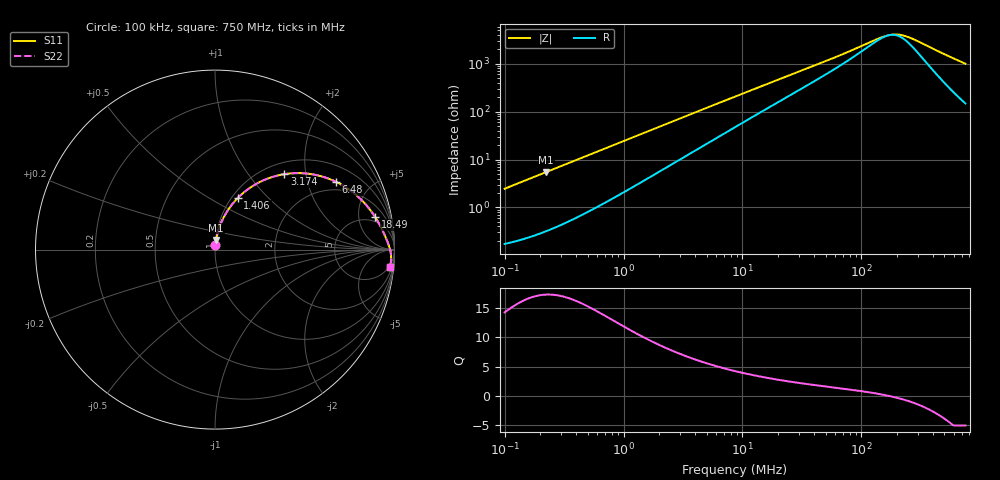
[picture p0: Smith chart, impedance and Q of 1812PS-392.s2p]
# MHz S MA R 50
!Freq  MagS11  AngS11  MagS21  AngS21  MagS12  AngS12  MagS22  AngS22
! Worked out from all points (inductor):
!   801 points, 100 kHz to 750 MHz, reference 50 ohm
!   read as one part in series: L = 3.89 uH near 104.6 kHz
!   highest Q = 17.2 at 223.2 kHz (marker M1), where L = 3.89 uH
!   self-resonance near 172.1 MHz
!   S11 on the Smith chart (normalised r, x): 100 kHz: 1.00, +0.05; 1.406 MHz: 1.07, +0.68; 3.174 MHz: 1.22, +1.52; 6.48 MHz: 1.62, +3.05; 18.49 MHz: 3.84, +8.16; 750 MHz: 4, -20
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0.1  0.02448 84.6  0.998 -1.4  0.998 -1.4  0.02448 84.6
0.2232315  0.05441 83.6  0.9954 -3.1  0.9954 -3.1  0.05441 83.6
0.4457309  0.1076 80.2  0.9874 -6.2  0.9874 -6.2  0.1076 80.2
0.8511669  0.2003 74.0  0.9641 -11.5  0.9641 -11.5  0.2003 74.0
1.406005  0.3148 66.1  0.9189 -18.3  0.9189 -18.3  0.3148 66.1
1.964725  0.4132 59.2  0.8649 -24.2  0.8649 -24.2  0.4132 59.2
2.539275  0.497 53.1  0.8064 -29.5  0.8064 -29.5  0.497 53.1
3.173849  0.5715 47.4  0.7432 -34.4  0.7432 -34.4  0.5715 47.4
4.484818  0.6797 38.3  0.6281 -42.1  0.6281 -42.1  0.6797 38.3
6.480241  0.7736 29.2  0.4975 -49.3  0.4975 -49.3  0.7736 29.2
8.660254  0.8285 23.0  0.401 -53.7  0.401 -53.7  0.8285 23.0
12.37465  0.8761 16.7  0.2994 -57.5  0.2994 -57.5  0.8761 16.7
18.48889  0.9107 11.5  0.2109 -59.3  0.2109 -59.3  0.9107 11.5
38.60143  0.9457 5.5  0.1074 -56.9  0.1074 -56.9  0.9457 5.5
71.28758  0.9617 2.6  0.05899 -48.2  0.05899 -48.2  0.9617 2.6
137.6574  0.9728 0.6  0.02911 -20.4  0.02911 -20.4  0.9728 0.6
170.1501  0.9754 0.0  0.02458 -1.2  0.02458 -1.2  0.9754 0.0
188.1164  0.9766 -0.2  0.02379 9.8  0.02379 9.8  0.9766 -0.2
205.673  0.9775 -0.5  0.02396 19.9  0.02396 19.9  0.9775 -0.5
248.6122  0.9793 -1.0  0.02703 39.4  0.02703 39.4  0.9793 -1.0
542.7381  0.9826 -3.8  0.06799 73.3  0.06799 73.3  0.9826 -3.8
750  0.981 -5.5  0.09734 76.0  0.09734 76.0  0.981 -5.5
